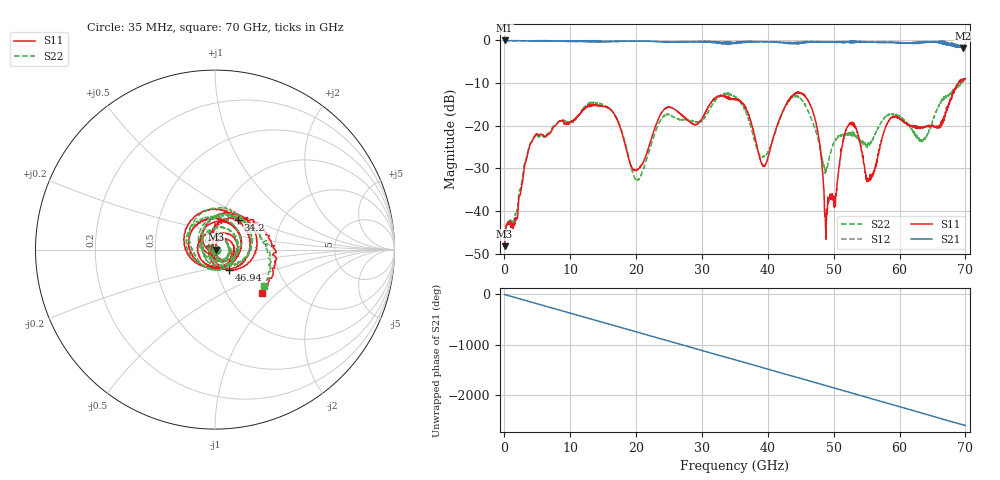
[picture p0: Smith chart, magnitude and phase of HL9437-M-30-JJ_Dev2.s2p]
! 7/27/2020 10:02:20 AM
! H:\PRODUCTION_DATA\TEMP_S2P.S2P
! CHANNEL.1
! TR.MEASUREMENT
! CORRECTED.DATA
# GHZ S RI R 50.0
! FREQ.GHZ  S11RE  S11IM  S21RE  S21IM  S12RE  S12IM  S22RE  S22IM
!; PortSelection: Port_12
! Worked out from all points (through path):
!   2000 points, 35 MHz to 70 GHz, reference 50 ohm
!   highest |S21| = -0.03 dB at 35 MHz (marker M1); lowest = -1.8 dB at 69.61 GHz (marker M2)
!   group delay of S21, straight-line fit = 104 ps
!   lowest |S11| = -48.2 dB at 35 MHz (marker M3), VSWR 1.01, Z = 50.4 - j0.115 ohm
!   |S11| at or under -10 dB: start of sweep to 68.96 GHz
!   |S22| runs from -48.2 to -9.3 dB; largest |S21 - S12| = 0.1
!   S11 on the Smith chart (normalised r, x): 35 MHz: 1.01, -0.00; 34.2 GHz: 1.22, +0.42; 46.94 GHz: 1.14, -0.27; 70 GHz: 1.45, -0.80
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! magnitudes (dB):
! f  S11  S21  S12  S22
! 35 MHz  -48.2  0.0  0.0  -48.2
! 1.715 GHz  -42.1  -0.1  -0.1  -41.0
! 4.48 GHz  -22.7  -0.2  -0.1  -22.8
! 11.72 GHz  -16.7  -0.2  -0.2  -16.6
! 16.48 GHz  -16.8  -0.3  -0.2  -16.9
! 20.12 GHz  -30.3  -0.2  -0.2  -32.8
! 23.38 GHz  -18.5  -0.3  -0.3  -19.8
! 34.2 GHz  -13.6  -0.8  -0.3  -12.7
! 35.03 GHz  -13.8  -0.5  -0.5  -13.2
! 39.38 GHz  -29.4  -0.3  -0.4  -27.2
! 43.68 GHz  -13.0  -0.6  -0.6  -13.4
! 46.69 GHz  -16.0  -0.4  -0.3  -18.7
! 46.94 GHz  -17.1  -0.4  -0.3  -19.9
! 48.93 GHz  -39.6  -0.4  -0.4  -29.7
! 50.23 GHz  -38.3  -0.4  -0.5  -23.6
! 52.19 GHz  -20.1  -0.4  -0.5  -21.7
! 55.34 GHz  -32.5  -0.4  -0.4  -24.0
! 58.34 GHz  -18.8  -0.5  -0.4  -17.5
! 63.52 GHz  -20.4  -0.4  -0.5  -23.6
! 66.22 GHz  -20.4  -0.4  -0.3  -14.5
! 69.61 GHz  -9.1  -1.8  -1.2  -9.8
! 70 GHz  -9.0  -1.3  -1.4  -9.4
